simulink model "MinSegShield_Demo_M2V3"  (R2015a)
settings: Solver=ode45  StartTime=0.0  StopTime=10.0  RelTol=1e-3
libraries: MinSegLibrary_M2V3 x11, arduinolib x5, RASPlib x1

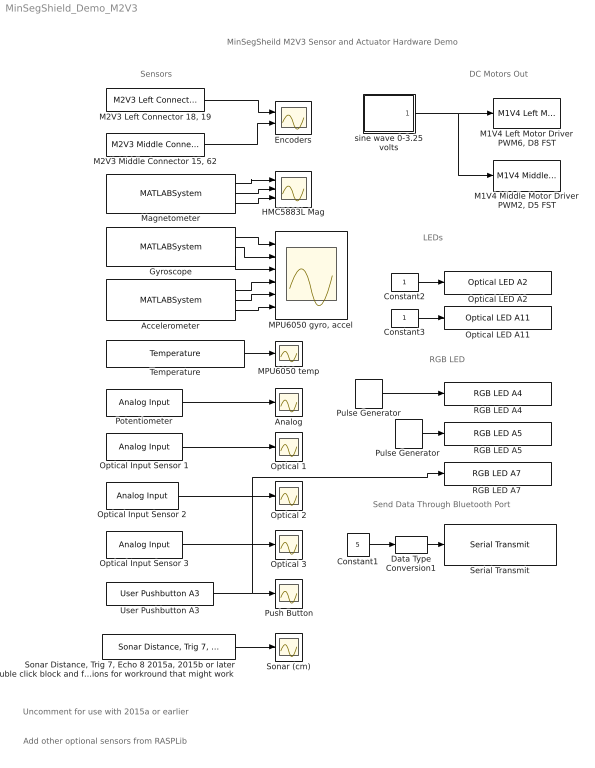
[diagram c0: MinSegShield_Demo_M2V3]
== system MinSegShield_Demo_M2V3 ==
  note: Send Data Through Bluetooth Port
  note: DC Motors Out
  note: Sensors
  note: MinSegSheild M2V3 Sensor and Actuator Hardware Demo
  note: LEDs
  note: RGB LED
  note: Uncomment for use with 2015a or earlier
  note: Add other optional sensors from RASPLib
  Accelerometer : MATLABSystem  System=soMPU6050Accel  SimulateUsing=Code generation
  Analog : Scope
  Constant1 : Constant  Value=5  SampleTime=-1
  Constant2 : Constant  SampleTime=-1
  Constant3 : Constant  SampleTime=-1
  Data Type Conversion1 : DataTypeConversion  OutDataTypeStr=uint8
  Encoders : Scope  NumInputPorts=2
  Gyroscope : MATLABSystem  System=soMPU6050Gyro  DLPFmode=0
  HMC5883L Mag : Scope  NumInputPorts=3
  "M1V4 Left Motor Driver PWM6, D8 FST" : MinSegLibrary_M2V3/M1V4 Left Motor Driver PWM6, D8 FST  Vsupply=3.25
  "M1V4 Middle Motor Driver PWM2, D5 FST" : MinSegLibrary_M2V3/M1V4 Middle Motor Driver PWM2, D5 FST  Vsupply=3.25
  "M2V3 Left Connector 18, 19" : MinSegLibrary_M2V3/M2V3 Left Connector 18, 19  Encoder=1  PinA=19  PinB=18
  "M2V3 Middle Connector 15, 62" : MinSegLibrary_M2V3/M2V3 Middle Connector 15, 62  Encoder=3  PinA=15  PinB=62
  "MPU6050 gyro, accel" : Scope  NumInputPorts=6
  MPU6050 temp : Scope
  Magnetometer : MATLABSystem  System=soHMC5883L  SimulateUsing=Code generation
  Optical 1 : Scope
  Optical 2 : Scope
  Optical 3 : Scope
  Optical Input Sensor 1 : arduinolib/Analog Input  pinNumber=10  sampleTime=-1  blockPlatform=arduino
  Optical Input Sensor 2 : arduinolib/Analog Input  pinNumber=1  sampleTime=-1  blockPlatform=arduino
  Optical Input Sensor 3 : arduinolib/Analog Input  pinNumber=9  sampleTime=-1  blockPlatform=arduino
  Optical LED A11 : MinSegLibrary_M2V3/Optical LED A11  Pin=11
  Optical LED A2 : MinSegLibrary_M2V3/Optical LED A2  Pin=2
  Potentiometer : arduinolib/Analog Input  pinNumber=0  sampleTime=-1  blockPlatform=arduino
  Pulse Generator : DiscretePulseGenerator  PulseType=Time based  Period=9  PulseWidth=50
  "Pulse Generator " : DiscretePulseGenerator  PulseType=Time based  Period=6  PulseWidth=50
  Push Button : Scope
  RGB LED A4 : MinSegLibrary_M2V3/RGB LED A4  Pin=4
  RGB LED A5 : MinSegLibrary_M2V3/RGB LED A5  Pin=5
  "RGB LED A7 " : MinSegLibrary_M2V3/RGB LED A7   Pin=7
  Serial Transmit : arduinolib/Serial Transmit  portNumber=2  blockPlatform=arduino
  Sonar (cm) : Scope
  "Sonar Distance, Trig 7, Echo 8 2015a, 2015b or later double click block and follow instructions for workround that might work" : MinSegLibrary_M2V3/Sonar Distance, Trig 7, Echo 8 2015a, 2015b or later double click block and follow instructions for workround that might work  Commented=on  TrigPin=12  EchoPin=11
  Temperature : RASPlib/Temperature  SimulateUsing=Code generation
  User Pushbutton A3 : MinSegLibrary_M2V3/User Pushbutton A3  Pin=3
  sine wave 0-3.25 volts : Subsystem
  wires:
  "M2V3 Left Connector 18, 19"/1 -> Encoders/1
  "M2V3 Middle Connector 15, 62"/1 -> Encoders/2
  "Sonar Distance, Trig 7, Echo 8 2015a, 2015b or later double click block and follow instructions for workround that might work"/1 -> Sonar (cm)/1
  Optical Input Sensor 1/1 -> Optical 1/1
  Constant1/1 -> Data Type Conversion1/1
  Data Type Conversion1/1 -> Serial Transmit/1
  Optical Input Sensor 2/1 -> Optical 2/1
  Optical Input Sensor 3/1 -> Optical 3/1
  Potentiometer/1 -> Analog/1
  Magnetometer/2 -> HMC5883L Mag/2
  Magnetometer/3 -> HMC5883L Mag/3
  Gyroscope/1 -> "MPU6050 gyro, accel"/1
  Gyroscope/2 -> "MPU6050 gyro, accel"/2
  Gyroscope/3 -> "MPU6050 gyro, accel"/3
  Accelerometer/3 -> "MPU6050 gyro, accel"/6
  Magnetometer/1 -> HMC5883L Mag/1
  sine wave 0-3.25 volts/1(sine) -> "M1V4 Middle Motor Driver PWM2, D5 FST"/1, "M1V4 Left Motor Driver PWM6, D8 FST"/1
  User Pushbutton A3/1 -> "RGB LED A7 "/1, Push Button/1
  Pulse Generator/1 -> RGB LED A4/1
  "Pulse Generator "/1 -> RGB LED A5/1
  Constant2/1 -> Optical LED A2/1
  Constant3/1 -> Optical LED A11/1
  Accelerometer/1 -> "MPU6050 gyro, accel"/4
  Accelerometer/2 -> "MPU6050 gyro, accel"/5
  Temperature/1 -> MPU6050 temp/1

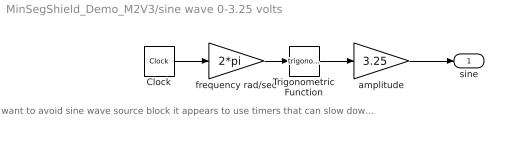
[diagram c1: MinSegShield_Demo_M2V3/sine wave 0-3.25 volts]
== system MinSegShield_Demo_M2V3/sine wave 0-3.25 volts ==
  note: want to avoid sine wave source block it appears to use timers that can slow down the serial port data transimission, and maybe other timers use a clock instead like this
  Clock : Clock
  Trigonometric Function : Trigonometry
  amplitude : Gain  Gain=3.25
  frequency rad/sec : Gain  Gain=2*pi
  sine : Outport
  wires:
  amplitude/1 -> sine/1
  frequency rad/sec/1 -> Trigonometric Function/1
  Trigonometric Function/1 -> amplitude/1
  Clock/1 -> frequency rad/sec/1
